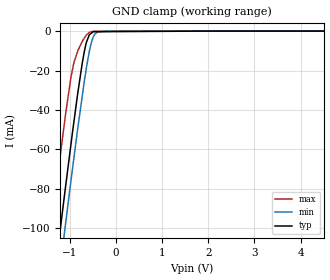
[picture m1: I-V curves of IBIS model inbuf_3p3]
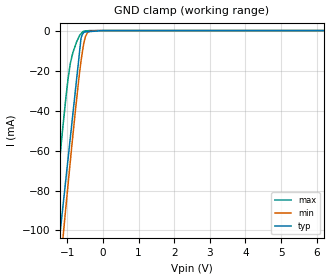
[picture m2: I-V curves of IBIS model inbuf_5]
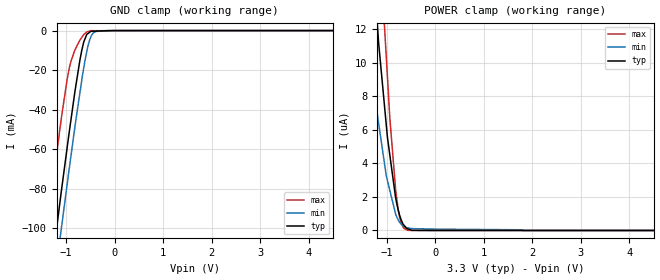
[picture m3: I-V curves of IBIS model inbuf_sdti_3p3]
|Texas Instruments Incorporated
|12-Channel, 16bit, Enhanced Spectrum PWM, RGB LED Driver
|   with 3.3V Linear Regulator and Watchdog Timer
| Marketing part#   Digital Voltage Range   Package-type   #pins
|   VREG
|TLC59711PWPR   3V to 5.5V   HTSSOP   20
|TLC59711PWP   3V to 5.5V   HTSSOP   20
|TLC59711RGER   3V to 5.5V   VQFN   24
|TLC59711RGET   3V to 5.5V   VQFN   24
[IBIS Ver]   4.0
[File name]   tlc59711.ibs
[File Rev]   1.0  |die revision A
|IBIS generated with SimDE V3.0 201101 Build 453
[Date]   07/27/2011
[Source]   Texas Instruments Incorporated.
   Analog-eLab, HPA
   12500 TI Blvd
   Dallas, TX -75243
   For Support e-mail: elab_ibis@list.ti.com
[Notes]   Revision History:
   1.0: 06/17/2011
   - Initial version of the model
   - Initial Model generated from simulations in TISPICED
   - Model names with a trailing _3p3 contains the model for
   3.3V (3.0V and 3.6V).
   _ Model names with trailing _5 contains
   the model for 5V (4.5V and 5.5V) operation.
   - Model not matched to measurements
   - C_comp although listed in numerical order of value are
   obtained from varying PVT conditions. For PVT conditions
   for each specific value refer the buffer description under
   respective [Model]. IBIS model user is responsible for using
   appropriate C_comp to simulate for Signal Integrity.
   2.0: 07/27/2011
   - Added t711_outbuf_1M_15p_3p3 and t711_outbuf_1M_15p_5 to model
   this buffer with a 1 Mohm and 15pF load. Buffers t711_outbuf_3p3
   and t711_outbuf_5 have a 50 ohm and 0pF load.
[Disclaimer]
  This model is designed as an aid for customers of Texas Instruments.
  TI and its licensors and suppliers make no warranties, either expressed
  or implied, with respect to this model, including the warranties of
  merchantability or fitness for a particular purpose.  The model is
  provided solely on an "as is" basis.  The entire risk as to its quality
  and performance is with the customer.
[Copyright] (C) Copyright 2011 Texas Instruments Incorporated.
   All rights reserved.
|   TLC59711
[Component]   tlc59711pwp
[Manufacturer] TI
[Package]   | 20 pin HTSSOP - PWP package
| variable   typ   min   max
R_pkg  8.87453E-02   6.79600E-02   1.16530E-01
L_pkg  2.46260nH   1.92739nH   3.29710nH
C_pkg  0.464608pF   0.418990pF   0.564180pF
|-------------------------PIN------------------------------------------------
[Pin] signal_name  model_name  R_pin  L_pin C_pin
1  IREF   TERM   0.09603  3.11915nH  0.55758pF
2  GND   GND   0.03723  2.26837nH  0.55786pF
3  OUTR0   TERM   0.08965  2.32165nH  0.43003pF
4  OUTG0   TERM   0.07489  2.05062nH  0.42686pF
5  OUTB0   TERM   0.06796  1.92739nH  0.41899pF
6  OUTR1   TERM   0.07201  2.00178nH  0.42375pF
7  OUTG1   TERM   0.08508  2.24016nH  0.43947pF
8  OUTB1   TERM   0.10300  2.57334nH  0.44718pF
9  SDTI   inbuf   0.11021  2.98985nH  0.51963pF
10 SCKI   inbuf_sdti   0.09557  3.12170nH  0.55478pF
11 SCKO   t711_outbuf  0.10515  3.29710nH  0.56418pF
12 SDTO   t711_outbuf  0.11653  3.10645nH  0.52794pF
13 OUTR2   TERM   0.10300  2.57334nH  0.44871pF
14 OUTG2   TERM   0.08508  2.24016nH  0.43960pF
15 OUTB2   TERM   0.07201  2.00178nH  0.42376pF
16 OUTR3   TERM   0.06796  1.92739nH  0.41900pF
17 OUTG3   TERM   0.07489  2.05062nH  0.42686pF
18 OUTB3   TERM   0.08965  2.32165nH  0.43001pF
19 VCC   TERM   0.08746  2.57356nH  0.49014pF
20 VREG   POWER   0.09336  3.07005nH  0.55148pF
[Component]   tlc59711rge
[Manufacturer] TI
[Package]   | 24 pin VQFN - RGE package
| variable   typ   min   max
R_pkg  7.17253E-02   5.54600E-02   8.45100E-02
L_pkg  1.25128nH   0.951090nH   1.49429nH
C_pkg  0.159139pF   0.142430pF   0.169790pF
|-------------------------PIN------------------------------------------------
[Pin] signal_name  model_name  R_pin  L_pin C_pin
1  SDTI   inbuf   0.07891  1.38979nH  0.15747pF
2  SCKI   inbuf_sdti   0.06270  1.08706nH  0.15151pF
3  NC   NC   0.00059  0.13682nH  0.09105pF
4  NC   NC   0.00059  0.13682nH  0.09104pF
5  SCKO   t711_outbuf  0.07055  1.22983nH  0.16009pF
6  SDTO   t711_outbuf  0.08451  1.49429nH  0.16505pF
7  OUTR2   TERM   0.08442  1.49159nH  0.16671pF
8  OUTG2   TERM   0.07470  1.30463nH  0.16979pF
9  OUTB2   TERM   0.06787  1.17732nH  0.16060pF
10 OUTR3   TERM   0.06521  1.12762nH  0.15699pF
11 OUTG3   TERM   0.06744  1.16743nH  0.15968pF
12 OUTB3   TERM   0.07396  1.29129nH  0.15126pF
13 VCC   TERM   0.06058  1.04800nH  0.13412pF
14 NC   NC   0.00059  0.13763nH  0.09099pF
15 VREG   POWER   0.05846  1.00333nH  0.14518pF
16 IREF   TERM   0.05546  0.95109nH  0.14243pF
17 NC   NC   0.00059  0.13763nH  0.09099pF
18 GND   GND   0.02321  0.83023nH  0.18416pF
19 OUTR0   TERM   0.07396  1.29129nH  0.15146pF
20 OUTG0   TERM   0.06744  1.16743nH  0.15972pF
21 OUTB0   TERM   0.06521  1.12762nH  0.15700pF
22 OUTR1   TERM   0.06787  1.17732nH  0.16058pF
23 OUTG1   TERM   0.07470  1.30463nH  0.16965pF
24 OUTB1   TERM   0.08442  1.49158nH  0.16537pF
|   Model Selectors
[Model Selector]  inbuf
inbuf_3p3   3.3V digital input
inbuf_5   5V digital input
|NOTES   Model inbuf split into two Models inbuf_3p3 and inbuf_5
|   to accomodate vast voltage range of 2.7V - 5.5V
|   inbuf_3p3 operates in voltage range of 3 - 3.3 - 3.6
|   inbuf_5 operates in voltage range of 4.5 - 5 - 5.5
|   The max pin frequency for Model inbuf is 20MHz.Also the
|   voltage range and frequency is referenced with datasheet.
[Model Selector]  inbuf_sdti
inbuf_sdti_3p3   3.3V digital input
inbuf_sdti_5   5V digital input
|NOTES   Model inbuf_sdti split into two Models inbuf_sdti_3p3 and
|   inbuf_sdti_5 to accomodate vast voltage range of 2.7V - 5.5V
|   inbuf_sdti_3p3 operates in voltage range of 3 - 3.3 - 3.6
|   inbuf_sdti_5 operates in voltage range of 4.5 - 5 - 5.5
|   The max pin frequency for Model inbuf_sdti is 10MHz.Also the
|   voltage range and frequency is referenced with datasheet.
[Model Selector]  t711_outbuf
t711_outbuf_3p3   3V digital output with 50 ohms and 0pf load
t711_outbuf_5   5V digital output with 50 ohms and 0pf load
t711_outbuf_IM_15p_3p3 with 1M ohms and 15pf load
t711_outbuf_IM_15p_5   with 1M ohms and 15pf load
|NOTES   Model t711_outbuf split into four Models t711_outbuf_3p3,
|   t711_outbuf_5, t711_outbuf_5, and t711_outbuf_5
|   to accomodate vast voltage range of 2.7V - 5.5V and two loads:
|   50 ohms / 0 pf and 1M ohms / 15 pF.
|   t711_outbuf_3p3 operates in voltage range of 3 - 3.3 - 3.6
|   with a load of 50 ohms and 0 pF.
|   t711_outbuf_5 operates in voltage range of 4.5 - 5 - 5.5
|   with a load of 50 ohms and 0 pF.
|   t711_outbuf_1M_15p_3p3 operates in voltage range of 3 - 3.3 - 3.6
|   with a load of 1M ohms and 15 pF.
|   t711_outbuf_1M_15p_5 operates in voltage range of 4.5 - 5 - 5.5
|   with a load of 1M ohms and 15 pF.
|   The max pin frequency for Model t711_outbuf is 10MHz.Also the
|   voltage range and frequency is referenced with datasheet.
[Model Selector]  TERM
TERM_3p3  3V digital output
TERM_5  5V digital output
|   TERM 3.3V Model
[Model] TERM_3p3
Model_type   Terminator
|   typ   min   max
|   (nom PVT)   (Fast PVT)   (slow PVT)
C_comp   1e-20   1e-20   1e-20
| Where   nom PVT is  Nominal Process, 3.3V, 90C
|   Fast PVT is Strong Process, 3.6V, -40C
|   Slow PVT is Weak Process, 3.0V, 150C
| variable   typ   min   max
[Voltage Range]   3.3   3   3.6
|Operating Temperature Range
|   25   85   -40
|Junction Temperature Range
[Temperature Range]   90   150   -40
|   TERM 5V Model
[Model] TERM_5
Model_type   Terminator
|   typ   min   max
|   (nom PVT)   (Fast PVT)   (slow PVT)
C_comp   1e-20   1e-20   1e-20
| Where   nom PVT is  Nominal Process, 5V, 90C
|   Fast PVT is Strong Process, 4.5V, -40C
|   Slow PVT is Weak Process, 5.5V, 150C
| variable   typ   min   max
[Voltage Range]   5   4.5   5.5
|Operating Temperature Range
|   25   85   -40
|Junction Temperature Range
[Temperature Range]   90   150   -40
| Models and submodels in the file (10): inbuf_3p3 (Input), inbuf_5 (Input), inbuf_sdti_3p3 (Input), inbuf_sdti_5 (Input), t711_outbuf_3p3 (Output), t711_outbuf_5 (Output), t711_outbuf_IM_15p_3p3 (Output), t711_outbuf_IM_15p_5 (Output), TERM_3p3 (Terminator), TERM_5 (Terminator)
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|NOTES   Model TERM split into two Models TERM_3p3 and
|   TERM_5 to accomodate vast voltage range of 2.7V - 5.5V
|   TERM_3p3 operates in voltage range of 3 - 3.3 - 3.6
|   TERM_5 operates in voltage range of 4.5 - 5 - 5.5
|   inbuf 3.3V Model
[Model] inbuf_3p3
Model_type   Input
Vinl = 0.99
Vinh = 2.31
|   typ   min   max
|   (nom PVT)   (Fast PVT)   (slow PVT)
C_comp   1.06189E-12   1.05216E-12   1.07666E-12
| Where   nom PVT is  Nominal Process, 3.3V, 90C
|   Fast PVT is Strong Process, 3.6V, -40C
|   Slow PVT is Weak Process, 3.0V, 150C
|   C_comp - from L-C Tank method, L = 1nH, peak frequency
[Model Spec]
|DVDD   3.3V   3.0V   3.6V
Vinl   0.99   0.9   1.08
Vinh   2.31   2.10   2.52
|Vinl   0.3 * VREG
|Vinh   0.7 * VREG
| variable   typ   min   max
[Voltage Range]   3.3   3   3.6
|Operating Temperature Range
|   25   85   -40
|Junction Temperature Range
[Temperature Range]   90   150   -40
[Power Clamp Reference]   3.3   3   3.6
[GND Clamp Reference]   0   0   0
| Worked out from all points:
|   GND clamp passes 1 mA (typ) near -0.53 V on its own axis
[GND Clamp]
|   Voltage   I(typ)   I(min)   I(max)
-3.3V     -514.2mA   -532.9mA   -476.6mA
-1.537V   -164.7mA   -183.8mA   -126.5mA
-1.303V   -119.4mA   -138.7mA   -81.63mA
-1.248V   -108.9mA   -128mA     -71.02mA
-1.151V   -90.55mA   -109.4mA   -53.44mA
-1.105V   -81.83mA   -100.7mA   -45.07mA
-907.1mV  -45.74mA   -64.04mA   -15.81mA
-717.6mV  -14.85mA   -31.21mA   -4.799mA
-571.2mV  -1.806mA   -9.88mA    -605.1uA
-455.6mV  -337.3uA   -1.542mA   -64.72uA
-164mV    -295.8uA   -5.21uA    -22.98uA
6.59V     0A         0A         0A
[POWER Clamp]
|   SCR cell for ESD function. Effects occurr above VDD x 2
|   Voltage   I(typ)   I(min)   I(max)
-3.3V     0A         0A         0A
0V        0A         0A         0A
6.6V      0A         0A         0A
|   inbuf 5V Model
[Model] inbuf_5
Model_type   Input
Vinl = 1.5
Vinh = 3.5
|   typ   min   max
|   (nom PVT)   (Fast PVT)   (slow PVT)
C_comp   9.61983E-13   9.55169E-13   9.81936E-13
| Where   nom PVT is  Nominal Process, 5V, 90C
|   Fast PVT is Strong Process, 4.5V, -40C
|   Slow PVT is Weak Process, 5.5V, 150C
|   C_comp - from L-C Tank method, L = 1nH, peak frequency
[Model Spec]
|DVDD   5V   4.5V   5.5V
Vinl   1.5   1.35   1.65
Vinh   3.5   3.15   3.85
|Vinl   0.3 * VREG
|Vinh   0.7 * VREG
| variable   typ   min   max
[Voltage Range]   5   4.5   5.5
|Operating Temperature Range
|   25   85   -40
|Junction Temperature Range
[Temperature Range]   90   150   -40
[Power Clamp Reference]   5   4.5   5.5
[GND Clamp Reference]   0   0   0
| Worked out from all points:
|   GND clamp passes 1 mA (typ) near -0.54 V on its own axis
[GND Clamp]
|   Voltage   I(typ)   I(min)   I(max)
-5V       -855.1mA   -873.7mA   -817.5mA
-1.427V   -143.7mA   -162.7mA   -105.3mA
-1.232V   -106.2mA   -124.7mA   -68.07mA
-1.13V    -89.3mA    -105.4mA   -49.36mA
-1.049V   -75.96mA   -90.18mA   -35.42mA
-912.6mV  -53.27mA   -64.96mA   -16.34mA
-747.1mV  -25.84mA   -35.95mA   -6.061mA
-614.7mV  -3.887mA   -15.35mA   -1.592mA
-539mV    -995.8uA   -6.549mA   -286uA
-429.5mV  -574.6uA   -929.6uA   -87.5uA
-165.4mV  -222uA     -5.4uA     -712nA
9.985V    0A         0A         0A
[POWER Clamp]
|   SCR cell for ESD function. Effects occurr above VDD x 2
|   Voltage   I(typ)   I(min)   I(max)
-3.3V     0A         0A         0A
0V        0A         0A         0A
6.6V      0A         0A         0A
|   inbuf_sdti 3.3V Model
[Model] inbuf_sdti_3p3
Model_type   Input
Vinl = 0.99
Vinh = 2.31
|   typ   min   max
|   (nom PVT)   (Fast PVT)   (slow PVT)
C_comp   1.07661E-12   1.0668E-12   1.07666E-12
| Where   nom PVT is  Nominal Process, 3.3V, 90C
|   Fast PVT is Strong Process, 3.6V, -40C
|   Slow PVT is Weak Process, 3.0V, 150C
|   C_comp - from L-C Tank method, L = 1nH, peak frequency
[Model Spec]
|DVDD   3.3V   3.0V   3.6V
Vinl   0.99   0.9   1.08
Vinh   2.31   2.10   2.52
|Vinl   0.3 * VREG
|Vinh   0.7 * VREG
| variable   typ   min   max
[Voltage Range]   3.3   3   3.6
|Operating Temperature Range
|   25   85   -40
|Junction Temperature Range
[Temperature Range]   90   150   -40
[Power Clamp Reference]   3.3   3   3.6
[GND Clamp Reference]   0   0   0
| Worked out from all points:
|   GND clamp passes 1 mA (typ) near -0.53 V on its own axis
[GND Clamp]
|   Voltage   I(typ)   I(min)   I(max)
-3.3V     -516.2mA   -534.7mA   -478.5mA
-1.544V   -166.7mA   -185.8mA   -128.4mA
-1.258V   -111.6mA   -130.4mA   -73.23mA
-1.131V   -87.08mA   -105.8mA   -49.93mA
-1.105V   -82.03mA   -100.9mA   -45.13mA
-937.9mV  -51.28mA   -69.77mA   -19.07mA
-715mV    -14.53mA   -30.95mA   -4.723mA
-637mV    -5.61mA    -18.59mA   -1.937mA
-569.8mV  -1.789mA   -9.772mA   -587.4uA
-441.1mV  -297.7uA   -1.163mA   -61.02uA
-159mV    -97.88uA   -4.551uA   -42.97uA
6.59V     0A         0A         0A
[POWER Clamp]
|   Voltage   I(typ)   I(min)   I(max)
-3.3V     53.06uA    37.47uA    68.15uA
-1.506V   25.25uA    15.65uA    42.12uA
-1.21V    12.86uA    7.184uA    21.92uA
-1.173V   11.28uA    6.436uA    19.6uA
-1.061V   7.791uA    4.222uA    12.76uA
-1.011V   6.259uA    3.246uA    10.3uA
-937.9mV  4.47uA     2.379uA    6.652uA
-819.5mV  1.95uA     982.3nA    2.448uA
-794mV    1.581uA    798.3nA    1.811uA
-706.6mV  640.2nA    384.9nA    445.9nA
-561.5mV  90.71nA    151.3nA    2.002nA
6.59V     0A         0A         0A
